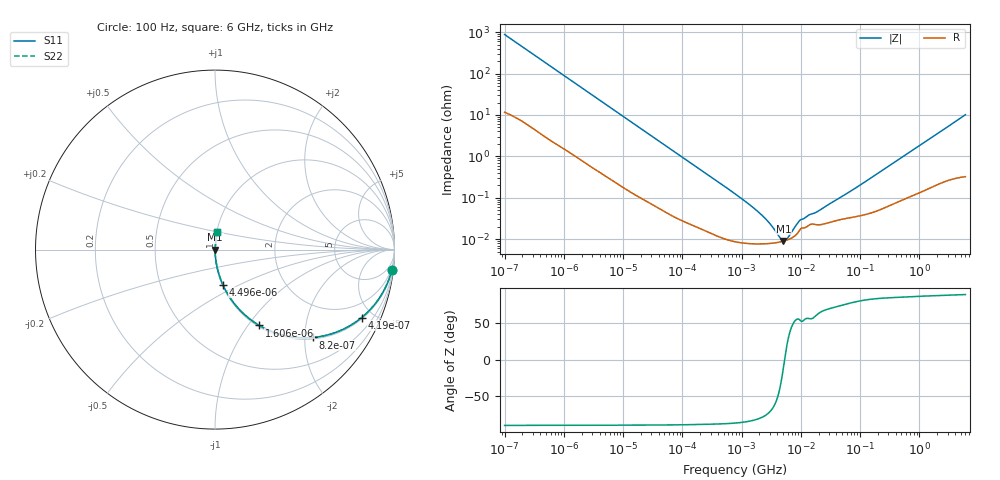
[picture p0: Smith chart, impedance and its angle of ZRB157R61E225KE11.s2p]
!Murata Part Number: ZRB157R61E225KE11
!These Parameters are Measured in Series Mode Connection
!Data Generated on Jun 10, 2025
!  o--ll--o
!Port1  Port2
!  o------o
!Operation Temp=25[degC], DC Bias Voltage=0[V]
!Freq. Start=100[Hz] Stop=6[GHz] 401[Steps]
# Hz S RI R 50
!Freq.(Hz) S11(Real) S11(Imag) S21(Real) S21(Imag) S12(Real) S12(Imag) S22(Real) S22(Imag)
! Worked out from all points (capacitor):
!   401 points, 100 Hz to 6 GHz, reference 50 ohm
!   read as one part in series: C = 1.8 uF near 109 Hz
!   lowest |Z| = 9.08 mohm at 5.079 MHz (marker M1)
!   series resonance near 5.325 MHz, so ESL is about 500 pH
!   S11 on the Smith chart (normalised r, x): 100 Hz: 1, -18; 419 Hz: 1.07, -4.28; 820 Hz: 1.04, -2.20; 1.606 kHz: 1.02, -1.13; 4.496 kHz: 1.01, -0.41; 6 GHz: 1.01, +0.20
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100  0.9859 -0.1115  0.0141 0.1115  0.0141 0.1115  0.9859 -0.1115
224  0.9373 -0.2346  0.0627 0.2346  0.0627 0.2346  0.9373 -0.2346
419  0.817 -0.3788  0.183 0.3788  0.183 0.3788  0.817 -0.3788
820  0.547 -0.4896  0.453 0.4896  0.453 0.4896  0.547 -0.4896
1122  0.3962 -0.4807  0.6038 0.4807  0.6038 0.4807  0.3962 -0.4807
1606  0.2467 -0.4225  0.7533 0.4225  0.7533 0.4225  0.2467 -0.4225
2008  0.1752 -0.3715  0.8248 0.3715  0.8248 0.3715  0.1752 -0.3715
4496  0.0434 -0.1949  0.9566 0.1949  0.9566 0.1949  0.0434 -0.1949
11514  0.008 -0.08  0.992 0.08  0.992 0.08  0.008 -0.08
40335  0.0011 -0.0234  0.9989 0.0234  0.9989 0.0234  0.0011 -0.0234
774597  8.79e-05 -0.00124  0.9999 0.00124  0.9999 0.00124  8.79e-05 -0.00124
2169299  7.68e-05 -0.00038  0.9999 0.00038  0.9999 0.00038  7.68e-05 -0.00038
3103719  7.9e-05 -0.00021  0.9999 0.00021  0.9999 0.00021  7.9e-05 -0.00021
4440638  8.51e-05 -6.78e-05  0.9999 6.78e-05  0.9999 6.78e-05  8.51e-05 -6.78e-05
5079039  8.91e-05 -1.75e-05  0.9999 1.75e-05  0.9999 1.75e-05  8.91e-05 -1.75e-05
6075234  9.69e-05 4.94e-05  0.9999 -4.94e-05  0.9999 -4.94e-05  9.69e-05 4.94e-05
9506416  0.000163 0.000226  0.9998 -0.000226  0.9998 -0.000226  0.000163 0.000226
1.555665e7  0.000231 0.000338  0.9998 -0.000338  0.9998 -0.000338  0.000231 0.000338
6.518806e7  0.000327 0.00133  0.9997 -0.00133  0.9997 -0.00133  0.000327 0.00133
3.124326e8  0.000676 0.00591  0.9993 -0.00591  0.9993 -0.00591  0.000676 0.00591
1.873145e9  0.00303 0.0326  0.997 -0.0326  0.997 -0.0326  0.00303 0.0326
6e9  0.0133 0.0998  0.9867 -0.0998  0.9867 -0.0998  0.0133 0.0998
